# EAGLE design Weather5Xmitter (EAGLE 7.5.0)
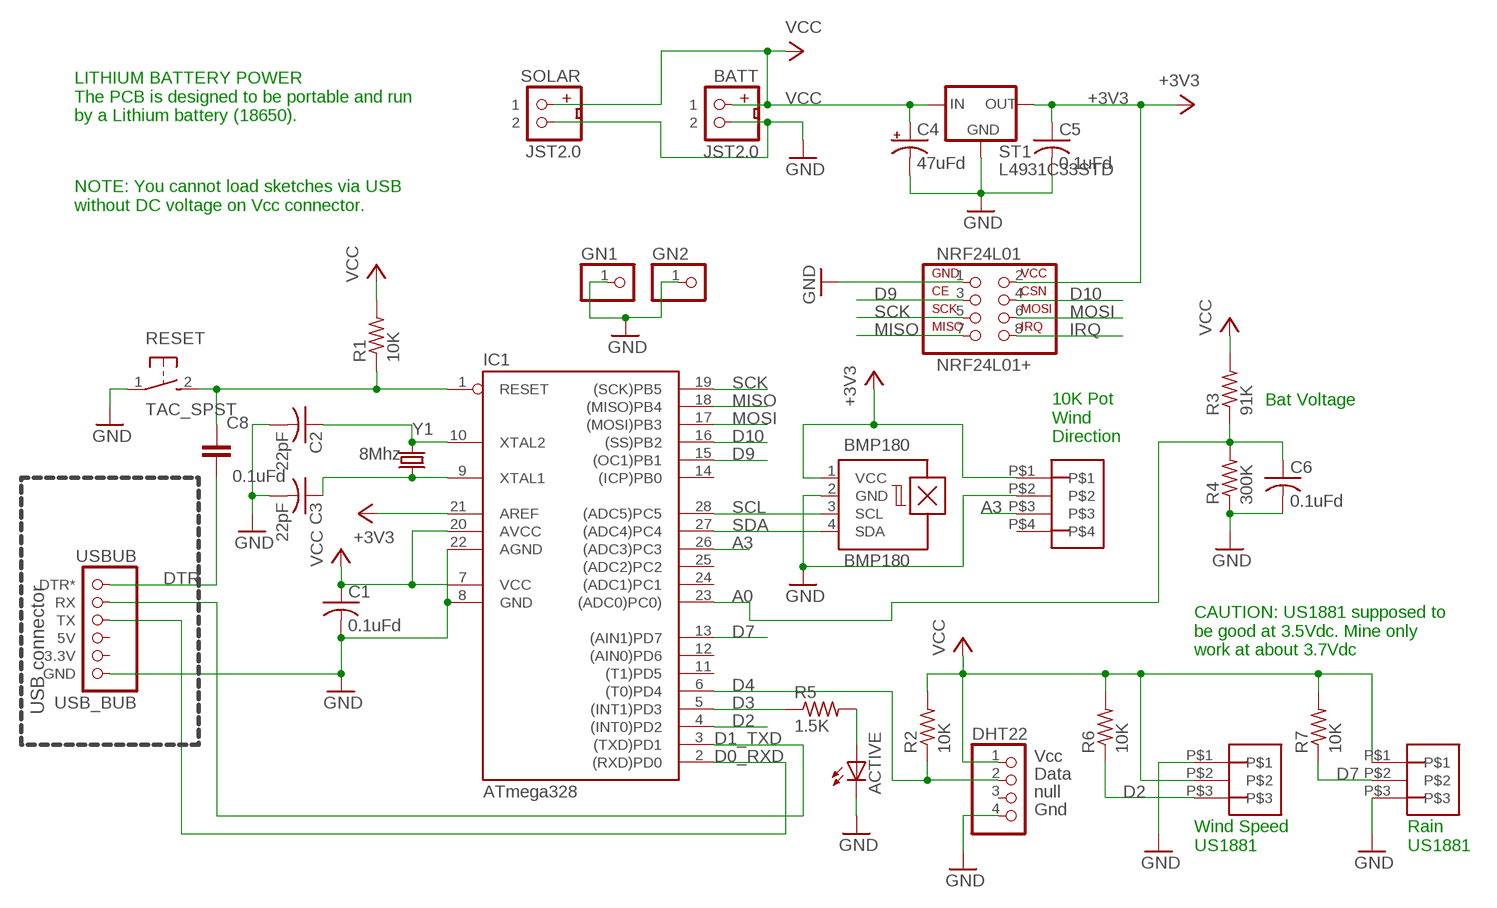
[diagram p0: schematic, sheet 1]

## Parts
ACTIVE  LED3MM  [LED3MM]
BATT  JST2.0  [JST2.0]
BMP180  BMP180  [BMP180]
C1  0.1uFd  C-US050-024X044  [C050-024X044]
C2  22pF  C-US025-025X050  [C025-025X050]
C3  22pF  C-US025-025X050  [C025-025X050]
C4  47uFd  CPOL-USE2.5-6  [E2,5-6]
C5  0.1uFd  C-US025-025X050  [C025-025X050]
C6  0.1uFd  C-US025-025X050  [C025-025X050]
C8  0.1uFd  C-EU075-032X103  [C075-032X103]
DHT22  DHT22  [1X04]
GN1  PINHD-1X1  [1X01]
GN2  PINHD-1X1  [1X01]
IC1  ATmega328  AT90S4433P  [DIL28-3]
NRF24L01  NRF24L01+  [NRF24L01+]
R1  10K  R-US_0207/2V  [0207/2V]
R2  10K  R-US_0207/2V  [0207/2V]
R3  91K  R-US_0204/7  [0204/7]
R4  300K  R-US_0207/2V  [0207/2V]
R5  1.5K  R-US_0207/2V  [0207/2V]
R6  10K  R-US_0207/7  [0207/7]
R7  10K  R-US_0207/10  [0207/10]
RAIN  3_PIN_JST-XH  [3_PIN_JST-XH]
RESET  TAC_SPST  [TACTILE-SPST]
SOLAR  JST2.0  [JST2.0]
ST1  L4931C33STD  [TO92-INLINE]
U$2  4_PIN_JST-XH  [4_PIN_JST-XH]
USBUB  USB_BUB  [USB_BUB]
WSPEED  3_PIN_JST-XH  [3_PIN_JST-XH]
Y1  8Mhz  CRYSTALTC38H  [TC38H]

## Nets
+3V3: BMP180.1(VCC) C5.1 IC1.21(AREF) NRF24L01.2 ST1.1(OUT) U$2.P$1
A0: C6.1 IC1.23((ADC0)PC0)) R3.1 R4.2
A3: IC1.26((ADC3)PC3) U$2.P$3
D0_RXD: IC1.2((RXD)PD0) USBUB.TX
D1_TXD: IC1.3((TXD)PD1) USBUB.RX
D2: IC1.4((INT0)PD2) R6.1 WSPEED.P$3
D3: IC1.5((INT1)PD3) R5.1
D4: DHT22.2(DATA) IC1.6((T0)PD4) R2.1
D7: IC1.13((AIN1)PD7) R7.1 RAIN.P$2
D9: IC1.15((OC1)PB1) NRF24L01.3
D10: IC1.16((SS)PB2) NRF24L01.4
DTR: C8.1 USBUB.DTR*
GND [power]: ACTIVE.K(C) BATT.2 BMP180.2(GND) C1.2 C2.2 C3.2 C4.- C5.2 C6.2 DHT22.4(GND) GN1.1 GN2.1 IC1.8(GND) IC1.22(AGND) NRF24L01.1 R4.1 RAIN.P$3 RESET.1 SOLAR.2 ST1.2(GND) U$2.P$2 USBUB.GND WSPEED.P$1
IRQ: NRF24L01.8
MISO: IC1.18((MISO)PB4) NRF24L01.7
MOSI: IC1.17((MOSI)PB3) NRF24L01.6
N$2: ACTIVE.A R5.2
N$4: C3.1 IC1.9(XTAL1) Y1.2
N$5: C2.1 IC1.10(XTAL2) Y1.1
RESET: C8.2 IC1.1(RESET) R1.1 RESET.2
SCK: IC1.19((SCK)PB5) NRF24L01.5
SCL: BMP180.3(SCL) IC1.28((ADC5)PC5)
SDA: BMP180.4(SDA) IC1.27((ADC4)PC4)
VCC: BATT.1 C1.1 C4.+ DHT22.1(VCC) IC1.7(VCC) IC1.20(AVCC) R1.2 R2.2 R3.2 R6.2 R7.2 RAIN.P$1 SOLAR.1 ST1.3(IN) WSPEED.P$2
Unconnected: DHT22.3(NULL) IC1.11((T1)PD5) IC1.12((AIN0)PD6) IC1.14((ICP)PB0) IC1.24((ADC1)PC1) IC1.25((ADC2)PC2) U$2.P$4 USBUB.3.3V USBUB.5V

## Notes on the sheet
- LITHIUM BATTERY POWER
  The PCB is designed to be portable and run
  by a Lithium battery (18650).
- NOTE: You cannot load sketches via USB 
  without DC voltage on Vcc connector.
- Bat Voltage
- 10K Pot
  Wind
  Direction
- CAUTION: US1881 supposed to 
  be good at 3.5Vdc. Mine only 
  work at about 3.7Vdc
- USB connector
- Wind Speed
  US1881
- Rain
  US1881

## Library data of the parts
ACTIVE = adafruit:LED: LED
BATT SOLAR = MTS_Custom:JST2.0: JST 2.0 2 pin connector 2mm spacing
BMP180 = MTS_Custom:BMP180
C1-C3 C5 C6 = MTS:C-US: CAPACITOR, American symbol
C4 = rcl:CPOL-US: POLARIZED CAPACITOR, American symbol
C8 = my-rcl:C-EU: CAPACITOR, European symbol
DHT22 = MTS_Custom:DHT22
GN1 GN2 = pinhead:PINHD-1X1: PIN HEADER
IC1 = atmel:AT90S4433: MICROCONTROLLER 4 Kbytes FLASH 128 bytes SRAM 256 bytes EEPROM UART 6-channel 10 bit ADC
NRF24L01 = MTS_Custom:NRF24L01+: 2.4GHz Transceiver
R1-R7 = MTS:R-US_: RESISTOR, American symbol
RAIN WSPEED = JST-XH_HEADERS:3_PIN_JST-XH
RESET = MTS_Custom:TAC_SPST: Tactile switch SPST 7mm lead spacing
ST1 = MTS_Custom:L4931C33: Voltage Regulator 3.3Vdc LDO (0.4V) 250mA output
U$2 = JST-XH_HEADERS:4_PIN_JST-XH
USBUB = MTS:USB_BUB
Y1 = MTS:CRYSTAL: Crystals

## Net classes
0 default: width 0.4 mm, clearance 0.3 mm
1 power: width 0.6 mm, clearance 0.3 mm

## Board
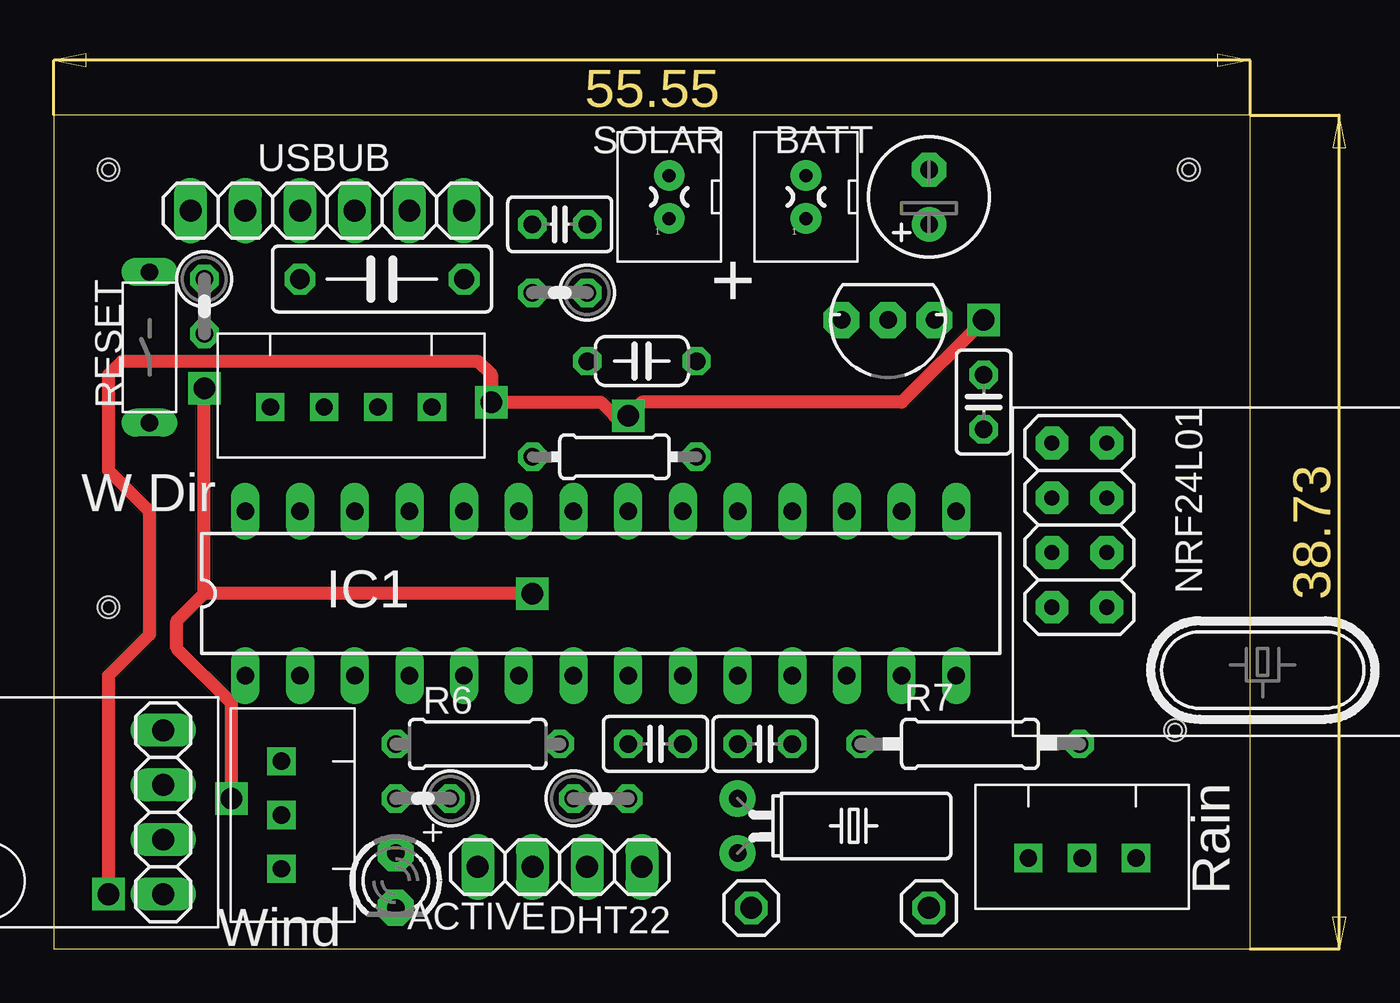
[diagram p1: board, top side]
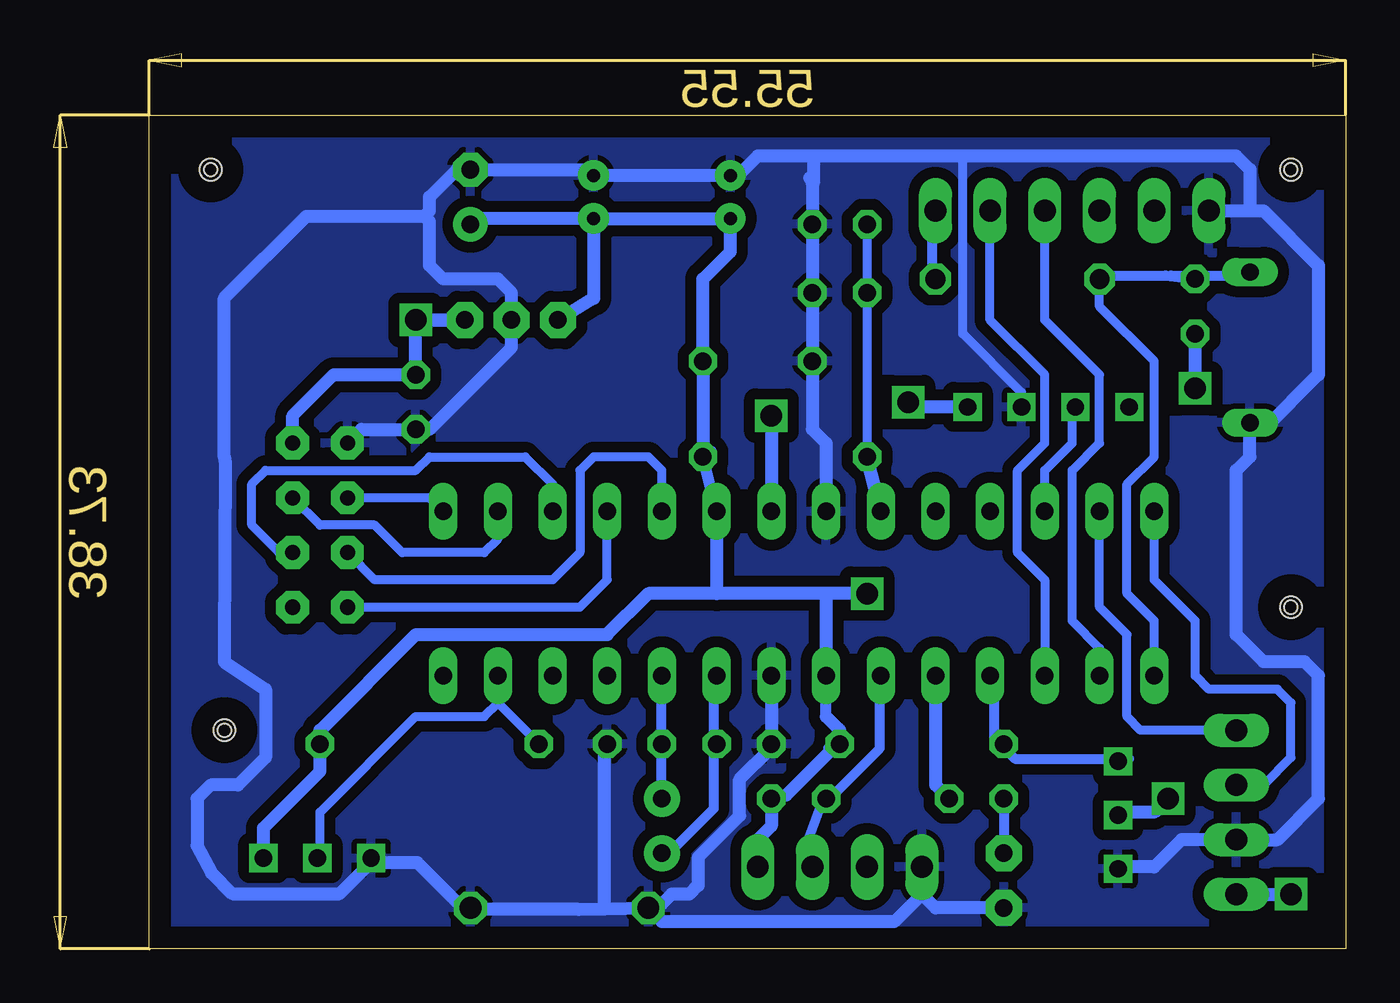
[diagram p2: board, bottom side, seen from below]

Size 59.99 x 41.57 mm. Coordinates in mm from the lower left corner, seen from the top.
Outline: 0,0 55.55,0 55.55,38.73 0,38.73 0,0
Copper layers (1*16): Top 0.035mm / dielectric 1.5mm / Bottom 0.035mm
Design rules "NewMTS": minimum track width 20mil, minimum drill 24mil, track to track 20mil, track to pad 20mil, pad to pad 8mil, via to via 8mil, smd to smd 8mil, copper to edge 40mil, drill to drill 8mil, minimum pad ring 10mil, minimum via ring 10mil, stop-mask expansion 4mil, vias tented up to drill 0mil, thermal gap 10mil
Holes 0.6 mm at 2.54,36.2 52.7,36.2 52.07,10.16 2.54,15.88
Holes 1 mm at 2.54,36.2 52.7,36.2 52.07,10.16 2.54,15.88

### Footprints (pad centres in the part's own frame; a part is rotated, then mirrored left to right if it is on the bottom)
LED3MM = drill 0.813 pad 1.676 octagon: A -1.27,0; K 1.27,0
JST2.0 = drill 0.6 pad 1.422: 1 0,-1; 2 0,1
BMP180 = drill 1.016 long: 1 -3.81,-1.27; 2 -1.27,-1.27; 3 1.27,-1.27; 4 3.81,-1.27
C050-024X044 = drill 0.813 octagon: 1 -2.54,0; 2 2.54,0
C025-025X050 = drill 0.813 octagon: 1 -1.27,0; 2 1.27,0
E2,5-6 = drill 0.813 pad 1.6: + -1.27,0 | drill 0.813 pad 1.6 octagon: - 1.27,0
C075-032X103 = drill 0.914 octagon: 1 -3.81,0; 2 3.81,0
1X04 = drill 1.016 long: 1 -3.81,0; 2 -1.27,0; 3 1.27,0; 4 3.81,0
1X01 = drill 1.016 octagon: 1 0,0
DIL28-3 = drill 0.813 long: 1 -16.51,-3.81; 2 -13.97,-3.81; 3 -11.43,-3.81; 4 -8.89,-3.81; 5 -6.35,-3.81; 6 -3.81,-3.81; 7 -1.27,-3.81; 8 1.27,-3.81; 9 3.81,-3.81; 10 6.35,-3.81; 11 8.89,-3.81; 12 11.43,-3.81; 13 13.97,-3.81; 14 16.51,-3.81; 15 16.51,3.81; 16 13.97,3.81; 17 11.43,3.81; 18 8.89,3.81; 19 6.35,3.81; 20 3.81,3.81; 21 1.27,3.81; 22 -1.27,3.81; 23 -3.81,3.81; 24 -6.35,3.81; 25 -8.89,3.81; 26 -11.43,3.81; 27 -13.97,3.81; 28 -16.51,3.81
NRF24L01+ = drill 0.7 pad 1.524 octagon: 1 -5.08,-12.7; 2 -5.08,-10.16; 3 -2.54,-12.7; 4 -2.54,-10.16; 5 0,-12.7; 6 0,-10.16; 7 2.54,-12.7; 8 2.54,-10.16
0207/2V = drill 0.813 octagon: 1 -1.27,0; 2 1.27,0
0204/7 = drill 0.813 octagon: 1 -3.81,0; 2 3.81,0
0207/7 = drill 0.813 octagon: 1 -3.81,0; 2 3.81,0
0207/10 = drill 0.813 octagon: 1 -5.08,0; 2 5.08,0
3_PIN_JST-XH = drill 0.8 square: P$1 2.45,3.4; P$2 4.95,3.4; P$3 7.45,3.4
TACTILE-SPST = drill 0.8 long: 1 0,3.5; 2 0,-3.5
TO92-INLINE = drill 0.813 pad 1.676 octagon: 1 -2.159,0; 2 0,0; 3 2.159,0
4_PIN_JST-XH = drill 0.8 square: P$1 2.45,3.4; P$2 4.95,3.4; P$3 7.45,3.4; P$4 9.95,3.4
USB_BUB = drill 1.016 long: 3.3V -3.81,0; 5V -1.27,0; DTR* 6.35,0; GND -6.35,0; RX 3.81,0; TX 1.27,0
TC38H = drill 0.813 pad 1.676: 1 -1.27,0; 2 1.27,0

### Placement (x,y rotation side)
ACTIVE  15.88,3.17 270 top
BATT  34.92,34.92 0 top
BMP180  3.81,6.35 90 top
C1  27.3,27.3 180 top
C2  33.02,9.53 0 top
C3  27.94,9.53 180 top
C4  40.64,34.92 90 top
C5  43.18,25.4 270 top
C6  23.5,33.66 0 top
C8  15.24,31.11 180 top
DHT22  23.5,3.81 180 top
GN1  32.38,1.91 0 top
GN2  40.64,1.91 0 top
IC1  25.4,16.51 0 top
NRF24L01  59.05,18.41 270 top
R1  6.99,29.84 270 top
R2  25.4,6.99 0 top
R3  26.04,22.86 0 top
R4  23.5,30.48 180 top
R5  17.14,6.99 180 top
R6  19.68,9.53 0 top
R7  42.55,9.53 0 top
RAIN  52.7,7.62 180 top
RESET  4.45,27.94 180 top
SOLAR  28.57,34.92 0 top
ST1  38.73,29.21 180 top
U$2  20,28.57 180 top
USBUB  12.7,34.29 0 top
WSPEED  13.97,1.27 90 top
Y1  31.75,5.71 270 top

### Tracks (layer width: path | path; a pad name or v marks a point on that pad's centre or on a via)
+3V3  (via drill 1)
  Top 0.61: v43.18,29.21 39.37,25.4 27.3,25.4 v26.67,24.77 26.04,24.77 25.4,25.4 v20.32,25.4 20.32,26.67 19.68,27.3 3.17,27.3 2.54,26.67 2.54,22.23 4.45,20.32 4.45,14.61 2.54,12.7 v2.54,2.54
  Bottom 0.406: NRF24L01.2 48.9,24.13
  Bottom 0.61: 48.9,24.13 48.9,24.77 46.99,26.67 C5.1 43.18,28.57 42.55,29.21 ST1.1 v43.18,29.21 | v26.67,24.77 IC1.21 | U$2.P$1 20.09,25.18 v20.32,25.4 | BMP180.1 v2.54,2.54
A0
  Bottom 0.406: C6.1 R4.2 R3.1
  Bottom 0.61: IC1.23 R3.1
A3
  Bottom 0.406: IC1.26 13.97,22.23 12.7,23.5 12.7,25.03 U$2.P$3
D0_RXD
  Bottom 0.406: IC1.2 11.43,13.97 12.7,15.24 12.7,22.23 11.43,23.5 11.43,26.67 13.97,29.21 USBUB.TX
D1_TXD
  Bottom 0.406: IC1.3 13.97,17.14 15.24,18.41 15.24,22.23 13.97,23.5 13.97,26.67 16.51,29.21 USBUB.RX
D2
  Bottom 0.457: WSPEED.P$3 10.05,8.84 15.35,8.84 15.84,9.32 R6.1 16.08,9.56 16.32,9.8 16.32,12.7 IC1.4
D3
  Bottom 0.61: IC1.5 19.05,7.62 R5.1
D4
  Bottom 0.457: DHT22.2 24.77,4.01 24.92,5.13 24.28,6.91 R2.1 24.04,6.91 21.63,9.32 21.63,12.7 IC1.6
D7
  Bottom 0.406: IC1.13 39.37,11.43 | 39.37,11.43 R7.1 | 47.62,4.35 47.62,6.35 43.18,10.79 40.01,10.79 39.37,11.43
  Bottom 0.508: RAIN.P$2 47.75,4.32 47.62,4.35
D9
  Bottom 0.406: IC1.15 42.55,20.95 NRF24L01.3
D10
  Bottom 0.406: IC1.16 39.37,19.05 40.01,18.41 43.81,18.41 45.09,19.68 47.62,19.68 NRF24L01.4
DTR
  Bottom 0.457: C8.1 19.21,31.28 19.21,34.18 USBUB.DTR*
GND
  Bottom 0.406: U$2.P$2 15.05,25.85 17.78,28.57 17.78,36.83
  Bottom 0.6: IC1.8 C3.2 26.7,9.32 28.14,7.87 28.14,6.18 30.07,4.25 | 34.41,1.86 35.62,1.84 40.45,1.84 GN2.1 40.93,1.84 43.1,4.01 45.03,4.01 RAIN.P$3 45.28,4.01 46.72,2.56 51.7,2.56 52.67,3.53 53.34,4.8 53.34,6.99 52.7,7.62 51.44,7.62 50.16,8.89 50.16,12.06 52.07,13.34 52.07,13.97 52.03,22.59 52.07,22.86 52.07,30.23 48.26,34.04 47.75,34.04 | 34.41,1.86 GN1.1 32.24,2.08 31.76,2.08 | C2.2 34.42,9.32 34.42,2.08 34.41,1.86 | 24.89,35.81 24.7,35.62
  Bottom 0.61: USBUB.GND 4.45,34.29 | 4.45,34.29 3.81,34.29 1.27,31.75 1.27,26.67 3.81,24.13 4.13,24.13 RESET.1 4.45,22.86 5.08,22.23 5.08,14.61 3.81,13.34 1.91,13.34 1.27,12.7 1.27,6.99 3.17,5.08 BMP180.2 7.62,5.08 8.89,3.81 10.48,3.81 WSPEED.P$1 | 24.77,36.83 17.78,36.83 5.08,36.83 4.45,36.2 4.45,34.29 | 24.77,36.83 27.3,36.83 28.21,35.92 SOLAR.2 BATT.2 35.2,36.2 C4.- 41.27,36.2 42.55,34.92 42.55,34.29 42.8,34.04 | 19.68,2.54 DHT22.4 | ACTIVE.K 19.05,1.91 19.68,2.54 | 19.68,2.54 20.95,1.27 31.75,1.27 GN1.1 | 30.07,4.25 30.07,2.95 30.48,2.54 31.3,2.54 31.76,2.08 | IC1.22 24.13,23.5 24.77,24.13 C1.2 R4.1 C6.2 24.77,35.56 24.7,35.62 24.7,36.77 24.77,36.83 | 47.75,34.04 42.8,34.04 | 42.8,34.04 42.55,33.78 42.55,31.75 41.91,31.11 39.37,31.11 38.73,30.48 ST1.2 38.73,27.94 42.55,24.13 C5.2 45.72,24.13 NRF24L01.1
  pour Bottom: 0,0 0,39.37 55.88,39.37 55.88,0
MISO
  Bottom 0.406: NRF24L01.7 35.56,15.88 34.29,17.14 IC1.18
MOSI
  Bottom 0.406: NRF24L01.6 49.53,18.41 50.8,19.68 50.8,21.59 50.16,22.23 43.18,22.23 42.55,22.86 38.1,22.86 36.83,21.59 IC1.17
N$2
  Bottom 0.457: R5.2 15.84,6.91 15.84,4.5 ACTIVE.A
N$4
  Bottom 0.457: IC1.9 29.35,12.7 29.35,9.56 C3.1 29.35,9.32 29.35,6.51 31.52,4.34 31.52,4.5 Y1.2
N$5
  Bottom 0.457: Y1.1 31.76,7.15 31.76,9.32 C2.1 31.76,9.56 31.76,12.7 IC1.10
RESET
  Bottom 0.406: IC1.1 8.89,15.24 10.16,16.51 10.16,21.59 8.89,22.86 8.89,27.3 11.43,29.84 C8.2
  Bottom 0.457: RESET.2 5.22,31.28 8.12,31.28 R1.1 8.36,31.28 11.25,31.28 C8.2
SCK
  Bottom 0.406: IC1.19 31.75,22.23 32.38,22.86 34.92,22.86 35.56,22.23 35.56,18.41 36.83,17.14 45.09,17.14 NRF24L01.5
SCL
  Bottom 0.406: BMP180.3 3.81,7.62 2.54,8.89 2.54,11.43 3.17,12.06 6.35,12.06 6.99,12.7 6.99,15.24 8.89,17.14 IC1.28
  Bottom 0.457: 8.84,20.18 IC1.28
SDA
  Bottom 0.406: BMP180.4 9.53,10.16 10.16,10.79 10.16,14.61 11.43,15.88 IC1.27
VCC  (via drill 1)
  Top 0.61: v8.26,6.99 8.26,11.43 5.71,13.97 5.71,15.24 6.99,16.51 | v22.23,16.51 6.99,16.51 | 6.99,16.51 v6.99,26.04
  Bottom 0.406: 27.3,5.08 DHT22.1
  Bottom 0.457: 24.04,12.46 IC1.7 | 25.97,7.15 26.45,7.15 | 24.04,9.32 23.92,9.2 23.8,9.32 23.56,9.32 R6.2 23.56,9.56
  Bottom 0.508: 24.13,10.79 IC1.7 | IC1.20 R3.2 29.46,23.11
  Bottom 0.61: 26.45,7.15 R2.2 26.67,5.71 27.3,5.08 | 25.97,7.15 23.92,9.2 | 23.56,9.56 23.56,10.22 | 23.56,10.22 24.13,10.79 | R6.2 23.5,10.16 23.56,10.22 | RAIN.P$1 50.26,5.62 47.62,8.26 R7.2 47.62,10.16 43.18,14.61 34.29,14.61 32.38,16.51 29.21,16.51 | BATT.1 40.37,33.92 C4.+ | R3.2 C1.1 29.84,31.11 28.57,32.38 SOLAR.1 BATT.1 | IC1.20 29.21,16.51 | 24.13,16.51 IC1.7 | 24.13,16.51 29.21,16.51 | v8.26,6.99 8.89,6.35 10.57,6.35 WSPEED.P$2 | v22.23,16.51 24.13,16.51 | v6.99,26.04 R1.2 | BATT.1 34.92,30.23 ST1.3

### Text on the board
tNames: + | W Dir | Rain | Wind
